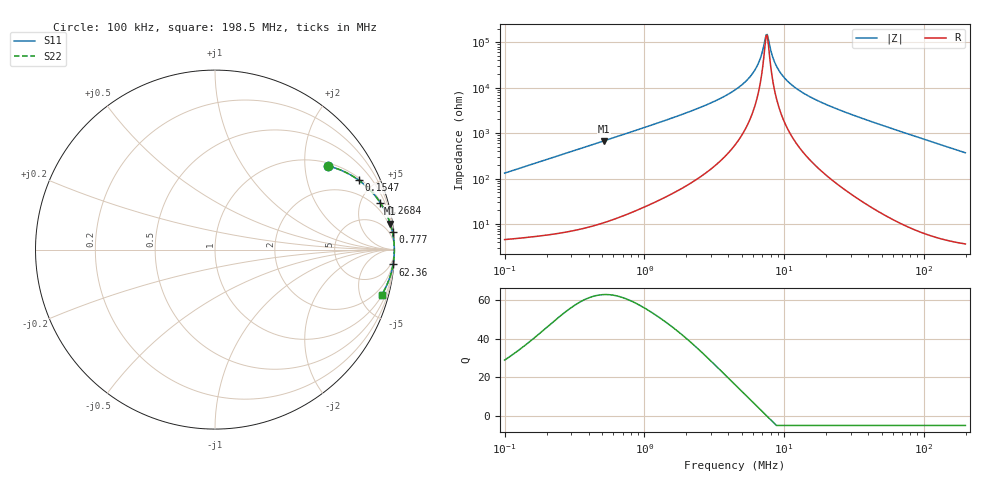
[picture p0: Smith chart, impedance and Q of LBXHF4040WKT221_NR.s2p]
! LBXHF4040WKT221_NR  S-PARAMETER MODEL  ( General Type )
! Model Generated by TAIYO YUDEN Corporation (http://www.ty-top.com)
! Version 1.0
! TAIYO YUDEN Control No. 210719NI43SB-FBB
! Copyright(c) 2021 TAIYO YUDEN CO.,LTD. All Rights Reserved.
! Product Description (link to TY-COMPAS)
! https://ds.yuden.co.jp/TYCOMPAS/or/detail?pn=LBXHF4040WKT221MNR&u=M
! Products Name : Inductors
! Characteristics :
!  Inductance : 220 uH , SRF(min) : 6.0 MHz , DC Resistance(max) : 3.36 Ohm
!  Rated Current : Saturation :330 mA , Temp Rise : 230 mA
!  Case Size : 4.0 x 4.0 / 0.157 x 0.157 [mm/inch] , Thickness : 2 / 0.079 [mm/inch]
!  (Conditions: Temperature = 25 degC , DC Bias Current/Voltage = 0A / 0V)
! External Node Assignments :
!  1  o---GGG---o  2
! GND o---------o GND
! Frequency Range : 0.1MHz  -  198.534594MHz  [ 402 STEP ]
# MHz S RI R 50
! Freq[MHz].  S11 Real  S11 Imag  S21 Real  S21 Imag  S12 Real  S12 Imag  S22 Real  S22 Imag
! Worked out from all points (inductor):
!   401 points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, 100 kHz to 198.5 MHz, reference 50 ohm
!   read as one part in series: L = 210 uH near 103.9 kHz
!   highest Q = 63 at 511.7 kHz (marker M1), where L = 210 uH
!   self-resonance near 7.439 MHz
!   S11 on the Smith chart (normalised r, x): 100 kHz: 1.09, +2.64; 154.7 kHz: 1.10, +4.08; 268.4 kHz: 1.13, +7.06; 777 kHz: 1, +21; 62.36 MHz: 1, -24; 198.5 MHz: 1.07, -7.41
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0.1  0.6319 0.4653  0.3681 -0.4653  0.3681 -0.4653  0.6319 0.4653
0.154748  0.8003 0.3872  0.1997 -0.3872  0.1997 -0.3872  0.8003 0.3872
0.268361  0.9217 0.2595  0.0783 -0.2595  0.0783 -0.2595  0.9217 0.2595
0.356769  0.9535 0.2023  0.0465 -0.2023  0.0465 -0.2023  0.9535 0.2023
0.511723  0.9763 0.1445  0.0237 -0.1445  0.0237 -0.1445  0.9763 0.1445
0.776991  0.9891 0.096  0.0109 -0.096  0.0109 -0.096  0.9891 0.096
1.272844  0.9955 0.0581  0.00453 -0.0581  0.00453 -0.0581  0.9955 0.0581
2.825192  0.9987 0.0233  0.00132 -0.0233  0.00132 -0.0233  0.9987 0.0233
4.541117  0.9992 0.0107  0.000804 -0.0107  0.000804 -0.0107  0.9992 0.0107
5.387211  0.9993 0.00694  0.000721 -0.00694  0.000721 -0.00694  0.9993 0.00694
6.152847  0.9993 0.00413  0.00068 -0.00413  0.00068 -0.00413  0.9993 0.00413
6.765487  0.9993 0.00216  0.000663 -0.00216  0.000663 -0.00216  0.9993 0.00216
7.299237  0.9993 0.000605  0.000655 -0.000605  0.000655 -0.000605  0.9993 0.000605
7.581701  0.9993 -0.000171  0.000653 0.000171  0.000653 0.000171  0.9993 -0.000171
7.727005  0.9993 -0.000559  0.000653 0.000559  0.000653 0.000559  0.9993 -0.000559
8.496385  0.9993 -0.00251  0.000656 0.00251  0.000656 0.00251  0.9993 -0.00251
9.7039  0.9993 -0.00527  0.000674 0.00527  0.000674 0.00527  0.9993 -0.00527
11.9574  0.9993 -0.00983  0.000741 0.00983  0.000741 0.00983  0.9993 -0.00983
15.89665  0.9991 -0.0168  0.000928 0.0168  0.000928 0.0168  0.9991 -0.0168
56.71438  0.9935 -0.0753  0.00651 0.0753  0.00651 0.0753  0.9935 -0.0753
62.36145  0.9922 -0.083  0.00777 0.083  0.00777 0.083  0.9922 -0.083
198.5346  0.9299 -0.2504  0.0701 0.2504  0.0701 0.2504  0.9299 -0.2504
